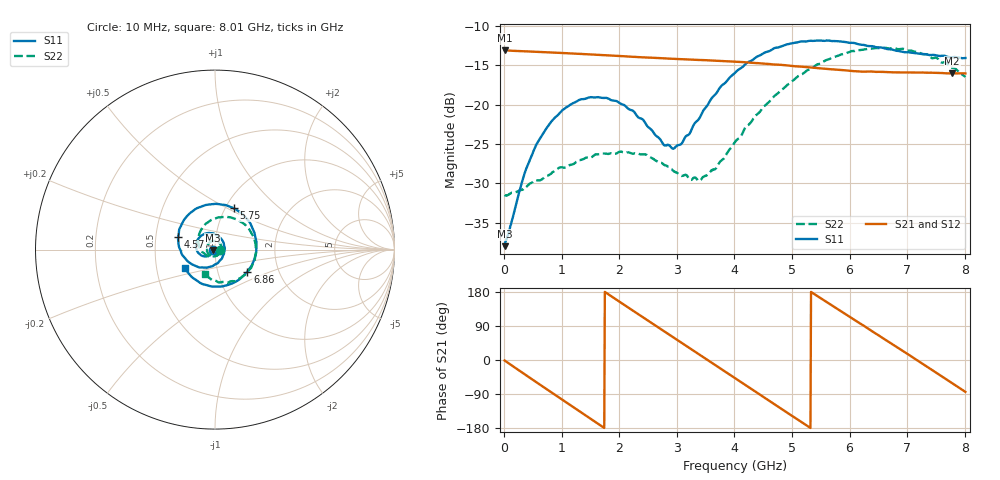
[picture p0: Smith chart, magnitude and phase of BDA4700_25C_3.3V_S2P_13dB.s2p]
!Agilent Technologies,E5071B,MY42404982,A.09.10
!Date: Mon Oct 20 18:08:29 2025
!Data & Calibration Information:
!Freq	S11:SOLT2(ON)	S21:SOLT2(ON)	S12:SOLT2(ON)	S22:SOLT2(ON)
# Hz S RI R 50
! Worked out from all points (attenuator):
!   801 points, 10 MHz to 8.01 GHz, reference 50 ohm
!   highest |S21| = -13.10 dB at 10 MHz (marker M1); lowest = -16.1 dB at 7.78 GHz (marker M2)
!   lowest |S11| = -38.0 dB at 10 MHz (marker M3), VSWR 1.03, Z = 48.8 - j0.156 ohm
!   |S11| at or under -10 dB: start of sweep to end of sweep
!   |S22| runs from -31.6 to -12.8 dB; largest |S21 - S12| = 0.0025
!   S11 on the Smith chart (normalised r, x): 10 MHz: 0.98, -0.00; 4.57 GHz: 0.65, +0.09; 5.75 GHz: 1.09, +0.54; 6.86 GHz: 1.39, -0.36; 8.01 GHz: 0.70, -0.15
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1e7  -0.0125 -0.0016  0.2212 -0.00486  0.2211 -0.005  0.0266 -0.000983
3.5e8  -0.0237 -0.0268  0.1744 -0.1303  0.1743 -0.1303  0.0222 -0.0189
5.7e8  -0.042 -0.0376  0.1096 -0.1861  0.1094 -0.186  0.0136 -0.0301
8.7e8  -0.0743 -0.0337  -0.00142 -0.2134  -0.00126 -0.2136  -0.00963 -0.0365
1.35e9  -0.1067 0.0175  -0.1593 -0.1358  -0.1593 -0.1359  -0.0423 -0.0139
1.94e9  -0.0577 0.0883  -0.192 0.0685  -0.192 0.0685  -0.0321 0.0366
2.33e9  0.00566 0.0827  -0.103 0.1714  -0.1031 0.1714  0.000629 0.0487
2.68e9  0.0471 0.04  0.0144 0.1967  0.014 0.1967  0.0281 0.0327
2.96e9  0.0513 -0.0126  0.1037 0.1649  0.1036 0.1646  0.0362 0.00979
3.39e9  0.00214 -0.0816  0.1855 0.0486  0.1858 0.0488  0.0194 -0.0263
3.67e9  -0.0587 -0.1001  0.1845 -0.0438  0.1846 -0.0443  -0.00756 -0.0383
4.01e9  -0.1407 -0.0737  0.1261 -0.1385  0.1264 -0.1381  -0.0483 -0.0313
4.57e9  -0.205 0.0688  -0.0445 -0.1756  -0.0441 -0.1759  -0.0925 0.0411
4.94e9  -0.1615 0.1803  -0.138 -0.1102  -0.1376 -0.1112  -0.0768 0.1111
5.35e9  -0.0395 0.2506  -0.1714 0.00687  -0.1715 0.00583  -0.00526 0.1698
5.75e9  0.104 0.2304  -0.1244 0.1108  -0.1242 0.111  0.0972 0.1765
6.23e9  0.2174 0.0992  -0.00528 0.1615  -0.00296 0.1616  0.2022 0.0933
6.68e9  0.2149 -0.0655  0.1081 0.1185  0.1085 0.1184  0.2246 -0.0323
6.86e9  0.1803 -0.1229  0.1381 0.0801  0.1385 0.0791  0.2084 -0.0835
7.31e9  0.0408 -0.2048  0.1544 -0.0395  0.1545 -0.0395  0.1181 -0.1716
7.78e9  -0.1171 -0.1619  0.0766 -0.1375  0.0765 -0.1377  -0.00823 -0.171
8.01e9  -0.1672 -0.1048  0.0162 -0.1566  0.0167 -0.1568  -0.0559 -0.1386
